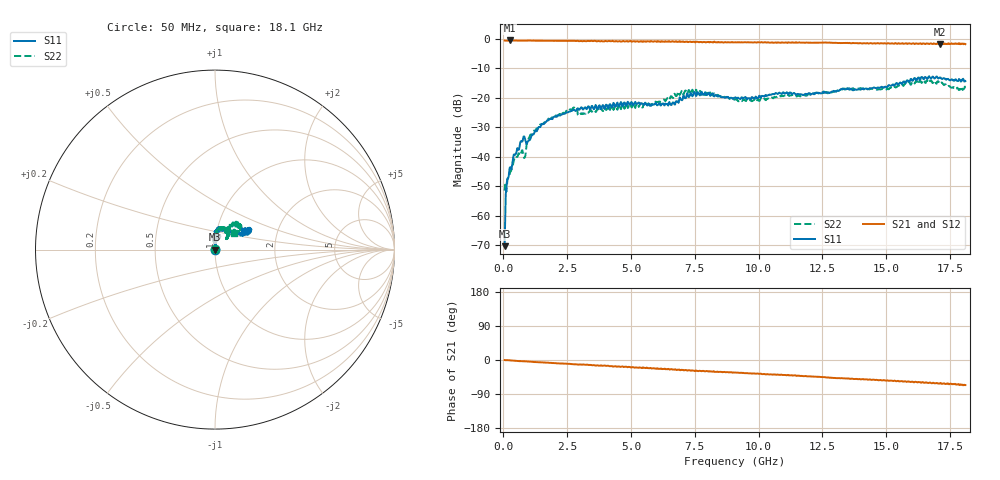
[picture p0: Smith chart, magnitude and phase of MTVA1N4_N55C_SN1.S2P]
! Network Analyzer HP8720D.06.14 Serial No. US36140669
! 12 Jan 2005  08:45:40
! Frequency  S11  S21  S12  S22
# HZ  S  DB R 50
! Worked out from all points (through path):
!   801 points, 50 MHz to 18.1 GHz, reference 50 ohm
!   highest |S21| = -0.51 dB at 253.1 MHz (marker M1); lowest = -1.8 dB at 17.11 GHz (marker M2)
!   group delay of S21, straight-line fit = 9.85 ps
!   lowest |S11| = -70.4 dB at 50 MHz (marker M3), VSWR 1.00, Z = 50 + j0.00395 ohm
!   |S11| at or under -10 dB: start of sweep to end of sweep
!   |S22| runs from -51.9 to -13.9 dB; largest |S21 - S12| = 0.031
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5e7  -70.40 7.5  -0.54 -0.1  -0.57 -0.5  -51.54 29.6
1.85375e8  -47.40 87.0  -0.55 -0.5  -0.55 -0.9  -47.17 70.3
2.530625e8  -43.68 90.0  -0.51 -1.0  -0.51 -1.5  -45.80 70.6
5.0125e8  -38.78 92.2  -0.54 -2.6  -0.54 -2.8  -40.27 81.2
7.494375e8  -34.84 84.4  -0.60 -3.2  -0.59 -3.6  -37.85 78.6
8.6225e8  -34.36 66.9  -0.59 -3.5  -0.57 -4.0  -39.67 115.5
1.087875e9  -33.35 87.6  -0.57 -4.8  -0.54 -4.8  -32.43 100.2
1.494e9  -28.93 86.4  -0.61 -6.3  -0.61 -6.5  -29.09 97.8
2.689812e9  -24.42 78.6  -0.64 -10.8  -0.65 -11.0  -23.92 99.0
3.073375e9  -23.30 77.0  -0.71 -12.3  -0.65 -12.5  -25.40 97.2
4.946062e9  -22.36 73.9  -0.76 -18.5  -0.72 -19.4  -21.86 91.2
6.074188e9  -22.32 79.6  -0.83 -23.5  -0.81 -23.3  -21.44 87.0
6.63825e9  -21.56 82.2  -0.81 -25.4  -0.84 -25.0  -20.07 81.2
7.202312e9  -18.47 82.2  -0.88 -27.7  -0.92 -27.2  -18.68 65.3
7.834062e9  -19.00 79.5  -1.03 -28.8  -0.99 -29.8  -18.05 53.1
9.075e9  -19.92 89.0  -1.15 -32.9  -1.07 -33.5  -20.56 43.9
1.209838e10  -18.67 65.8  -1.26 -43.7  -1.23 -43.9  -18.63 58.1
1.331675e10  -16.93 48.4  -1.38 -48.4  -1.36 -48.4  -16.94 59.7
1.509919e10  -15.67 34.1  -1.48 -54.9  -1.39 -54.6  -17.08 58.5
1.61145e10  -13.26 28.2  -1.74 -58.1  -1.47 -58.2  -15.12 51.1
1.710725e10  -13.15 30.9  -1.81 -61.3  -1.71 -61.5  -15.31 40.0
1.81e10  -14.31 31.8  -1.75 -66.2  -1.74 -67.4  -16.94 40.5
